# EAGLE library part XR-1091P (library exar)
Equalizer FILTER
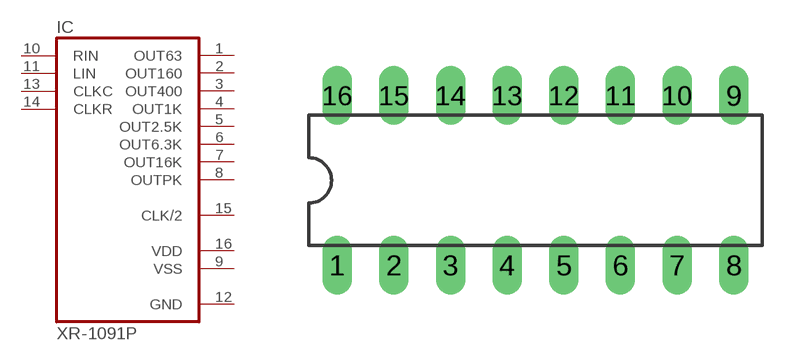
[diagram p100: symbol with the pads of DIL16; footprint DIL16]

Designator prefix IC

## XR-1091P (OC_FARNELL: unknown; OC_NEWARK: unknown)  [DIL16]
1  OUT63  out
2  OUT160  out
3  OUT400  out
4  OUT1K  out
5  OUT2.5K  out
6  OUT6.3K  out
7  OUT16K  out
8  OUTPK  out
9  VSS  pwr
10  RIN  in
11  LIN  in
12  GND  pwr
13  CLKC  in
14  CLKR  in
15  CLK/2  out
16  VDD  pwr

## Footprint DIL16 (pad centres in mm)
Dual In Line Package
drill 0.813 long: 1 -8.89,-3.81; 2 -6.35,-3.81; 3 -3.81,-3.81; 4 -1.27,-3.81; 5 1.27,-3.81; 6 3.81,-3.81; 7 6.35,-3.81; 8 8.89,-3.81; 9 8.89,3.81; 10 6.35,3.81; 11 3.81,3.81; 12 1.27,3.81; 13 -1.27,3.81; 14 -3.81,3.81; 15 -6.35,3.81; 16 -8.89,3.81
